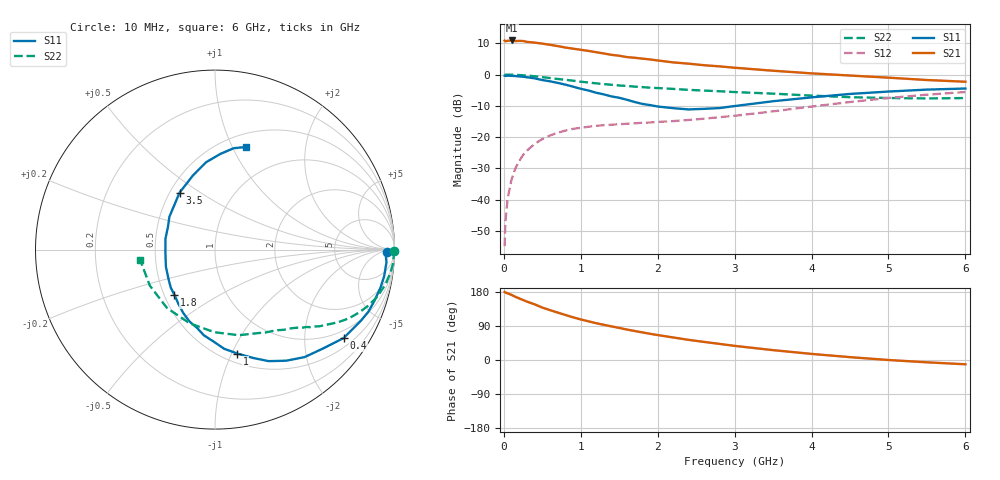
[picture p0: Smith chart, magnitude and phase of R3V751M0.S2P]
! SIEMENS Small Signal Semiconductors
! BFR181
! Si NPN RF Bipolar Junction Transistor in SOT23
! VCE = 0.75 V  IC = 1 mA
! Common Emitter S-Parameters:  May  1996
# GHz  S  MA  R  50
!  f  S11  S21  S12  S22
! GHz  MAG  ANG  MAG  ANG  MAG  ANG  MAG  ANG
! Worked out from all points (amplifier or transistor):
!   36 points, 10 MHz to 6 GHz, reference 50 ohm
!   highest |S21| = 10.9 dB at 100 MHz (marker M1)
!   |S21| within 3 dB of that: start of sweep to 1.006 GHz
!   unconditionally stable (mu >= 1): 1.898 GHz to 4.106 GHz
!   at 250 MHz: K = 0.17, MSG = 18.2 dB, |S12| = -25.7 dB
!   at 1.4 GHz: K = 0.81, MSG = 11.2 dB, |S12| = -16.0 dB
!   at 6 GHz: K = 0.94, MSG = 1.6 dB, |S12| = -5.6 dB
!   S11 on the Smith chart (normalised r, x): 10 MHz: 42, -16; 400 MHz: 0.75, -3.05; 1 GHz: 0.59, -1.05; 1.8 GHz: 0.57, -0.32; 3.5 GHz: 0.56, +0.41; 6 GHz: 0.64, +1.13
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0.01  0.9591 -0.9  3.495 179.5  0.0018 86.6  0.9982 -0.4
0.02  0.9519 -1.8  3.402 178.2  0.0044 86.1  0.9938 -0.9
0.05  0.9581 -4.2  3.462 175.9  0.0105 87.4  0.9964 -2.2
0.1  0.9541 -8.9  3.507 171.8  0.021 84.1  0.9953 -4.4
0.15  0.946 -13.0  3.425 166.7  0.0316 80.5  0.9881 -6.7
0.25  0.9222 -22.0  3.437 158.3  0.0518 74.9  0.9721 -10.9
0.3  0.904 -26.1  3.332 154.1  0.0607 73.1  0.9609 -12.8
0.4  0.8699 -34.5  3.239 146.9  0.0779 68.0  0.9389 -16.5
0.5  0.8159 -42.5  3.121 138.3  0.093 63.4  0.909 -20.1
0.6  0.7796 -50.2  2.989 131.6  0.106 58.9  0.8788 -23.3
0.8  0.6897 -64.3  2.703 118.8  0.1271 52.2  0.8229 -28.4
1  0.5921 -77.9  2.489 107.1  0.1408 46.9  0.7685 -32.5
1.1  0.555 -84.7  2.386 102.1  0.1462 44.9  0.745 -34.3
1.2  0.5113 -91.1  2.275 97.1  0.1511 43.0  0.7231 -36.2
1.4  0.4462 -103.2  2.065 88.6  0.1576 40.6  0.6852 -39.1
1.8  0.3389 -131.8  1.796 72.8  0.1692 39.3  0.6292 -43.8
2.2  0.2897 -160.8  1.564 59.5  0.18 39.9  0.5891 -49.3
2.8  0.2908 154.4  1.352 42.6  0.2076 43.3  0.5405 -58.7
3.5  0.3741 121.8  1.15 26.0  0.2578 44.7  0.4948 -74.6
4.5  0.4895 95.8  0.964 7.5  0.3634 40.0  0.4343 -109.0
5.5  0.5742 79.6  0.817 -6.1  0.4762 28.0  0.4149 -151.0
6  0.5976 73.2  0.767 -11.3  0.5249 20.5  0.4205 -171.9
